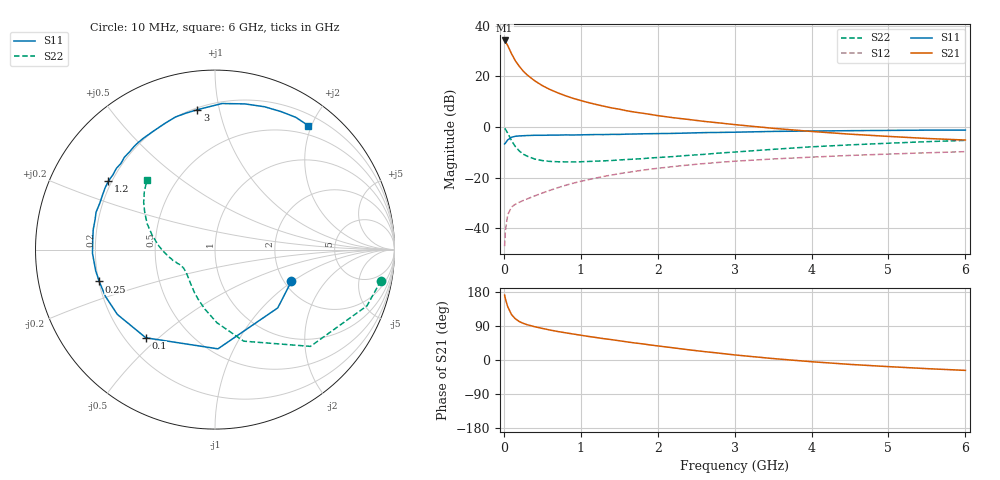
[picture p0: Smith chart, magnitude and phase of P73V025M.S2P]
! SIEMENS Small Signal Semiconductors
! BFP196
! Si NPN RF Bipolar Junction Transistor in SOT143
! VCE = 3 V  IC = 25 mA
! Common Emitter S-Parameters:  May  1996
# GHz  S  MA  R  50
!  f  S11  S21  S12  S22
! GHz  MAG  ANG  MAG  ANG  MAG  ANG  MAG  ANG
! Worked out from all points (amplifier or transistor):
!   36 points, 10 MHz to 6 GHz, reference 50 ohm
!   highest |S21| = 34.2 dB at 10 MHz (marker M1)
!   |S21| within 3 dB of that: start of sweep to 65.5 MHz
!   unconditionally stable (mu >= 1): 592 MHz to 3.432 GHz
!   at 250 MHz: K = 0.68, MSG = 25.6 dB, |S12| = -29.1 dB
!   at 1.4 GHz: K = 1.11, MAG = 11.3 dB, |S12| = -19.0 dB
!   at 6 GHz: K = 0.97, MSG = 2.3 dB, |S12| = -9.8 dB
!   S11 on the Smith chart (normalised r, x): 10 MHz: 2.18, -0.98; 100 MHz: 0.28, -0.45; 250 MHz: 0.20, -0.13; 1.2 GHz: 0.19, +0.28; 3 GHz: 0.21, +0.86; 6 GHz: 0.36, +1.95
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0.01  0.4608 -22.6  51.07 171.4  0.0044 83.5  0.9406 -10.6
0.02  0.4772 -42.9  48.55 161.8  0.0088 74.8  0.9028 -20.3
0.05  0.5531 -88.3  40.62 140.8  0.0183 59.4  0.7573 -45.4
0.1  0.6244 -128.1  27.9 119.8  0.0261 46.7  0.5346 -72.6
0.15  0.653 -146.4  20.26 108.6  0.0297 43.3  0.4075 -88.5
0.2  0.6639 -156.9  15.79 101.6  0.0324 43.4  0.3358 -99.8
0.25  0.6688 -164.6  12.78 96.9  0.035 44.1  0.2904 -109.1
0.3  0.6752 -169.9  10.76 93.3  0.0376 45.8  0.2653 -115.5
0.4  0.6828 -178.2  8.174 87.9  0.0433 48.6  0.2322 -126.1
0.5  0.6828 176.4  6.544 83.4  0.0493 52.0  0.2159 -133.5
0.6  0.6876 170.7  5.477 79.1  0.0559 53.6  0.208 -138.8
0.7  0.6883 166.3  4.715 75.2  0.0628 54.9  0.2049 -143.0
0.9  0.692 158.1  3.671 68.6  0.0771 55.4  0.2027 -149.2
1.1  0.7022 150.7  3.022 62.2  0.0907 55.1  0.2076 -153.3
1.2  0.7061 147.2  2.775 59.3  0.0978 55.0  0.2107 -155.4
1.6  0.721 134.4  2.081 47.8  0.1257 51.2  0.227 -161.5
2.2  0.7443 117.2  1.521 32.2  0.1644 44.5  0.2591 -170.7
3  0.7856 97.2  1.11 13.4  0.2101 34.0  0.3187 175.2
3.5  0.8147 87.3  0.939 3.8  0.2324 27.6  0.3605 166.8
4.5  0.8423 70.9  0.719 -11.6  0.273 16.1  0.4414 152.4
5.5  0.8636 58.6  0.591 -22.8  0.3081 5.3  0.5109 140.4
6  0.8645 53.1  0.55 -27.4  0.3244 -0.5  0.5413 134.4
